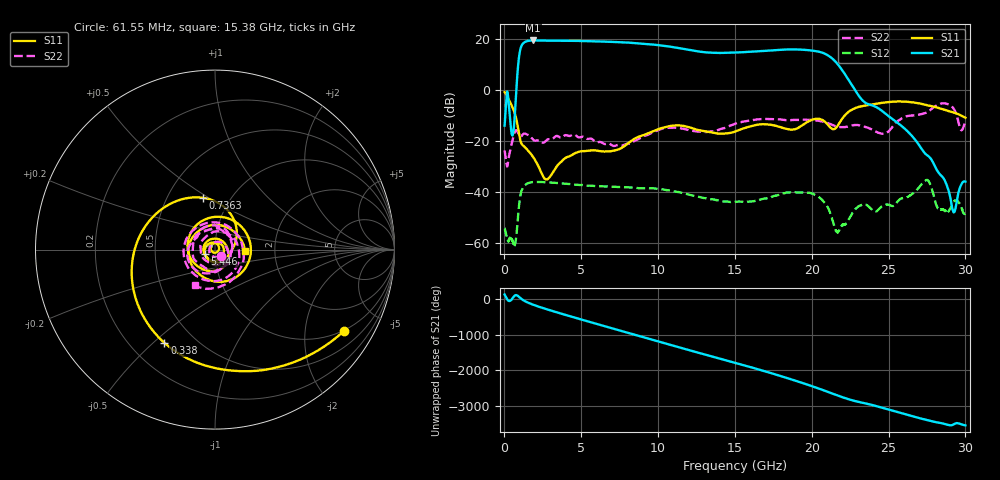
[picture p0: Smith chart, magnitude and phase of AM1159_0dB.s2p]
!Keysight Technologies,N5245B,MY58422270,A.16.20.02
!Date: Tuesday, December 10, 2024 22:46:40
!Correction: S11(C  2-Port  )
!S21(C  2-Port  )
!S12(C  2-Port  )
!S22(C  2-Port  )
!S2P File: Measurements: S11, S21, S12, S22:
# Hz S  dB  R 50
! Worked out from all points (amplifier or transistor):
!   6401 points, 10 MHz to 30 GHz, reference 50 ohm
!   highest |S21| = 19.3 dB at 1.875 GHz (marker M1)
!   |S21| within 3 dB of that: 1.055 GHz to 11.37 GHz (10.31 GHz wide, 166 % of centre)
!   unconditionally stable (mu >= 1): start of sweep to end of sweep
!   at 5.005 GHz: K = 4.09, MAG = 19.2 dB, |S12| = -37.4 dB
!   at 15.01 GHz: K = 13.70, MAG = 14.8 dB, |S12| = -43.9 dB
!   at 30 GHz: K = 7374.09, MAG = -35.4 dB, |S12| = -48.6 dB
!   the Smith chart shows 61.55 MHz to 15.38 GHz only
!   S11 on the Smith chart (normalised r, x): 61.55 MHz: 0.98, -3.20; 338 MHz: 0.34, -0.54; 736.3 MHz: 0.75, +0.47; 5.446 GHz: 0.89, -0.05; 15.38 GHz: 1.40, -0.02
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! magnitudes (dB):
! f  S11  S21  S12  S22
! 10 MHz  -0.9  -14.1  -54.3  -23.8
! 61.55 MHz  -1.4  -9.2  -55.5  -26.1
! 338 MHz  -4.6  -9.6  -58.2  -24.8
! 539.5 MHz  -7.2  -17.7  -59.4  -19.4
! 736.3 MHz  -10.6  -3.7  -59.1  -16.0
! 1.088 GHz  -20.9  16.8  -40.1  -18.3
! 1.875 GHz  -26.5  19.3  -36.2  -19.6
! 2.747 GHz  -35.2  19.2  -36.3  -19.8
! 5.01 GHz  -24.1  19.1  -37.4  -18.5
! 5.446 GHz  -23.9  19.0  -37.6  -19.3
! 7.639 GHz  -22.8  18.5  -38.2  -22.0
! 10.01 GHz  -15.5  17.4  -38.9  -15.8
! 15.01 GHz  -16.4  14.5  -43.9  -13.4
! 15.38 GHz  -15.6  14.6  -43.8  -12.8
! 20 GHz  -11.8  15.3  -40.7  -11.9
! 21.65 GHz  -14.4  10.2  -55.7  -14.5
! 23.15 GHz  -6.6  -3.1  -45.4  -14.0
! 25 GHz  -4.9  -10.4  -45.1  -16.4
! 27.46 GHz  -6.0  -25.5  -35.4  -9.0
! 28.28 GHz  -7.2  -32.7  -46.8  -5.7
! 29.23 GHz  -9.0  -48.0  -43.9  -7.4
! 30 GHz  -11.0  -36.0  -48.6  -12.5
